(* Logix 5000 AddOnInstructionDefinition export D_ROTR; software revision 17.00 *)

ADD_ON_INSTRUCTION D_ROTR   (* revision 2.0 20180219, vendor Kenneth A. Fischer *)
// DINT circular right shift (rotation) of the 32-bit argument Inp_A by Inp_B bits
// Revision note:
// Rev2.0: 20180219 - Corrected an error where an Inp_B = 0 results in no output being generated
// Rev1.0: 20170524 - Initial Release
VAR_IN_OUT
   Inp_A : DINT; {required}   // 64-bit Integer to be right circular rotated
END_VAR
VAR_INPUT
   Inp_B : INT; {required}   // Number of Inp_A bit rotations
END_VAR
VAR_IN_OUT
   Out : DINT; {required}   // Result
END_VAR
VAR
   Wrk_InpA : DINT[2];
   BSR_Cntrl : CONTROL := (LEN := 32);
   Source_Bit : BOOL;
   ONS : BOOL;
END_VAR

ROUTINE Logic   (* ladder *)
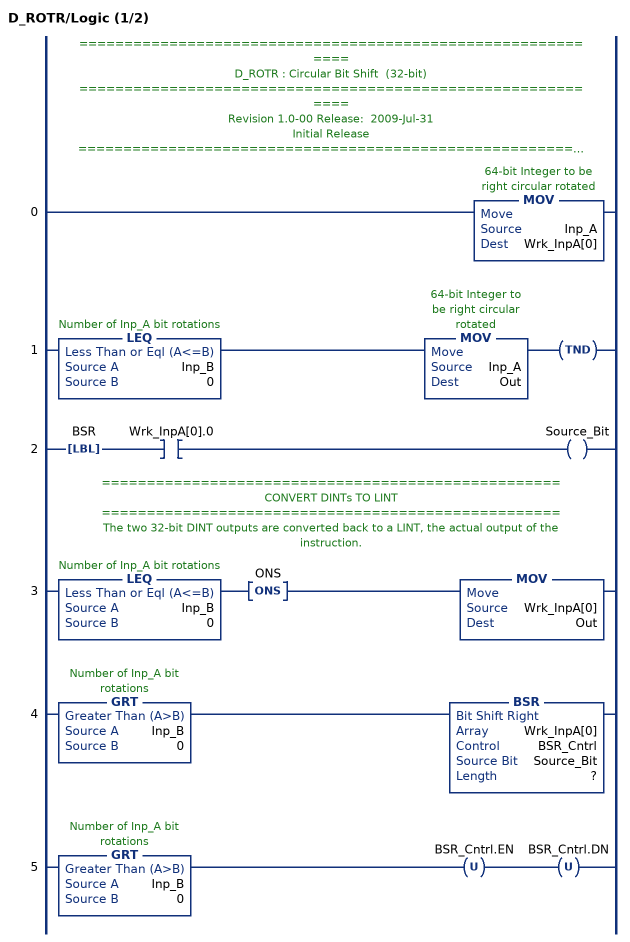
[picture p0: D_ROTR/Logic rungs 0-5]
   // ============================================================
   // D_ROTR : Circular Bit Shift  (32-bit)
   // ============================================================
   // Revision 1.0-00 Release:  2009-Jul-31
   // Initial Release
   // ============================================================
   // Performs a circular right shift rotation of the 32-bit argument Inp_A by the
   // number of bits defined in the 16-bit argument Inp_B.
   0: MOV(Inp_A,Wrk_InpA[0]);
   1: LEQ(Inp_B,0)MOV(Inp_A,Out)TND();
   2: LBL(BSR)XIC(Wrk_InpA[0].0)OTE(Source_Bit);
   // ===================================================
   // CONVERT DINTs TO LINT
   // ===================================================
   // The two 32-bit DINT outputs are converted back to a LINT, the actual output of the instruction.
   3: LEQ(Inp_B,0)ONS(ONS)MOV(Wrk_InpA[0],Out);
   4: GRT(Inp_B,0)BSR(Wrk_InpA[0],BSR_Cntrl,Source_Bit,?);
   5: GRT(Inp_B,0)OTU(BSR_Cntrl.EN)OTU(BSR_Cntrl.DN);
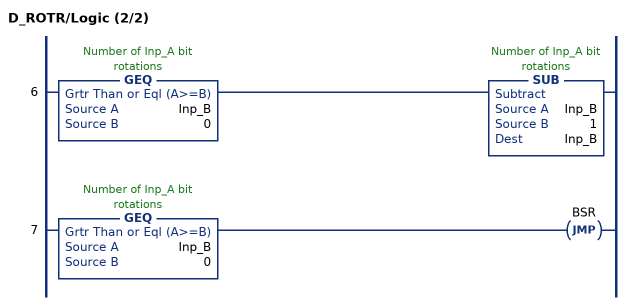
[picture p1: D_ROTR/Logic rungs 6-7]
   6: GEQ(Inp_B,0)SUB(Inp_B,1,Inp_B);
   7: GEQ(Inp_B,0)JMP(BSR);
END_ROUTINE
END_ADD_ON_INSTRUCTION
